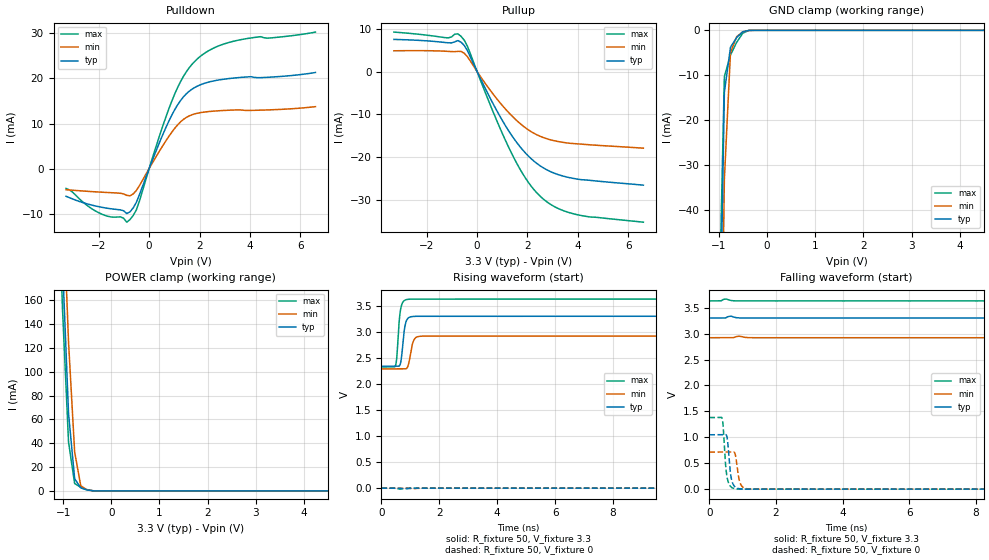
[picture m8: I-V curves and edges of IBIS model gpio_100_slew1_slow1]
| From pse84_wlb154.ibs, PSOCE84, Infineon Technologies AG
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[Model] gpio_100_slew1_slow1
Model_type I/O
Enable   Active-High
Vinl  =  0.99
Vinh  =  2.31
Vmeas =  1.65
Cref  =  15e-12
| Capacitance   typ   min   max
C_comp   1.09946e-12   1.08623e-12   1.11440e-12
| Variables   typ   min   max
[GND Clamp Reference]   0   0   0
[POWER Clamp Reference]   3.3   2.92   3.63
[Pulldown Reference]   0   0   0
[Pullup Reference]   3.3   2.92   3.63
[Temperature Range]   25   125   -40
[Voltage Range]   3.3   2.92   3.63
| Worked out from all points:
|   slope of the pulldown table from 0 to 0.495 V, typ, clamps not added: 71.6 ohm
|   slope of the pullup table from 0 to 0.495 V, typ, clamps not added: 83.3 ohm
|   GND clamp passes 1 mA (typ) near -0.57 V on its own axis
|   POWER clamp passes 1 mA (typ) near -0.52 V on its own axis
|   falling waveform, R_fixture 50, V_fixture 3.3: 20-80 % time 694ns typ, 1.01us min, 397ns max; typ from 3.3 V to 2.34 V
|   falling waveform, R_fixture 50, V_fixture 0: 20-80 % time 96.8ps typ, 105ps min, 93.7ps max; typ from 1.05 V to 0 V
|   rising waveform, R_fixture 50, V_fixture 3.3: 20-80 % time 114ps typ, 134ps min, 103ps max; typ from 2.34 V to 3.3 V
|   rising waveform, R_fixture 50, V_fixture 0: 20-80 % time 754ns typ, 1.06us min, 489ns max; typ from 0 V to 1.04 V
[GND Clamp]
| Voltage   I(typ)   I(min)   I(max)
-1.65V    -892.5mA   -911.9mA   -883.9mA
-1.015V   -92.32mA   -129.7mA   -71.28mA
-888.3mV  -13.83mA   -33.21mA   -10.31mA
-761.4mV  -3.792mA   -4.944mA   -5.509mA
-634.5mV  -1.622mA   -1.436mA   -2.707mA
-507.6mV  -326.2uA   -352.3uA   -651.6uA
-380.7mV  -13.48uA   -32.14uA   -19.55uA
-253.8mV  -189.4nA   -1.276uA   -466.7nA
6.6V      0A         0A         0A
[POWER Clamp]
| Voltage   I(typ)   I(min)   I(max)
-1.523V   838.1mA    872.9mA    823.9mA
-1.142V   346.5mA    405.1mA    310.5mA
-1.015V   193mA      257.4mA    153.9mA
-888.3mV  64.97mA    124.9mA    40.96mA
-761.4mV  10.28mA    32.7mA     6.184mA
-634.5mV  2.553mA    4.346mA    3.067mA
-507.6mV  805.9uA    960.7uA    1.159mA
-253.8mV  1.454uA    10.02uA    1.678uA
6.6V      0A         0A         0A
[Pulldown]
| Voltage   I(typ)   I(min)   I(max)
-3.3V     -6.15mA    -4.695mA   -4.423mA
-2.157V   -8.273mA   -5.161mA   -9.338mA
-1.142V   -9.173mA   -5.494mA   -10.74mA
-888.3mV  -9.988mA   -5.953mA   -11.91mA
-507.6mV  -7.509mA   -4.873mA   -9.177mA
341.4mV   4.84mA     3.249mA    6.058mA
910.3mV   11.98mA    8.158mA    15.13mA
1.366V    15.94mA    10.93mA    20.51mA
1.821V    18.03mA    12.15mA    23.86mA
2.503V    19.39mA    12.72mA    26.59mA
3.3V      20.06mA    12.98mA    28.19mA
6.6V      21.33mA    13.74mA    30.3mA
[Pullup]
| Voltage   I(typ)   I(min)   I(max)
-3.3V     7.527mA    4.862mA    9.247mA
-1.142V   6.736mA    4.723mA    7.893mA
-761.4mV  7.259mA    4.727mA    8.836mA
-634.5mV  6.867mA    4.72mA     8.248mA
-380.7mV  4.868mA    3.47mA     5.906mA
682.8mV   -8.07mA    -5.639mA   -10.11mA
1.479V    -15.86mA   -10.96mA   -20.44mA
2.048V    -19.88mA   -13.73mA   -26.08mA
2.731V    -22.92mA   -15.68mA   -30.37mA
3.3V      -24.31mA   -16.5mA    -32.32mA
4.051V    -25.28mA   -16.98mA   -33.65mA
6.6V      -26.63mA   -17.96mA   -35.32mA
[Ramp]
dV/dt_r   0.62586/0.754243u  0.420968/1.05896u  0.827993/0.488885u
dV/dt_f   0.573974/0.693875u  0.373545/1.01125u  0.781638/0.397055u
R_load = 50
[Falling Waveform]
R_fixture = 50
V_fixture = 3.3
V_fixture_min = 2.92
V_fixture_max = 3.63
| Time   V(typ)   V(min)   V(max)
0s        3.3V       2.92V      3.63V
127.1ns   3.3V       2.92V      3.598V
237.2ns   3.276V     2.92V      3.261V
319.8ns   3.185V     2.915V     3.022V
482.7ns   2.964V     2.86V      2.716V
645.6ns   2.788V     2.764V     2.553V
849.2ns   2.638V     2.653V     2.452V
1.282us   2.472V     2.492V     2.368V
1.92us    2.386V     2.378V     2.336V
4us       2.343V     2.297V     2.327V
[Falling Waveform]
R_fixture = 50
V_fixture = 0
V_fixture_min = 0
V_fixture_max = 0
| Time   V(typ)   V(min)   V(max)
0s        1.049V     715.3mV    1.381V
383.3ps   1.049V     715.1mV    1.364V
414.9ps   1.049V     715.1mV    1.21V
474.6ps   1.051V     715.2mV    568.4mV
511.4ps   1.041V     715.3mV    313.9mV
673.3ps   165mV      715.8mV    29.7mV
774.5ps   41.14mV    675mV      6.364mV
884.2ps   9.65mV     211.7mV    1.632mV
956.3ps   3.65mV     74.51mV    804.4uV
4us       19.97nV    549.4nV    10.01nV
[Rising Waveform]
R_fixture = 50
V_fixture = 3.3
V_fixture_min = 2.92
V_fixture_max = 3.63
| Time   V(typ)   V(min)   V(max)
0s        2.342V     2.29V      2.327V
480.6ps   2.341V     2.29V      2.345V
532.5ps   2.342V     2.29V      2.528V
626.9ps   2.352V     2.29V      3.285V
687ps     2.488V     2.29V      3.498V
780.9ps   3.002V     2.29V      3.598V
841.4ps   3.18V      2.291V     3.617V
931.3ps   3.268V     2.37V      3.626V
1.119ns   3.297V     2.841V     3.629V
4us       3.3V       2.92V      3.63V
[Rising Waveform]
R_fixture = 50
V_fixture = 0
V_fixture_min = 0
V_fixture_max = 0
| Time   V(typ)   V(min)   V(max)
0s        17.41nV    537.5nV    10.27nV
146.4ns   1.058mV    143.2uV    59.16mV
253.4ns   43.81mV    2.628mV    320.9mV
375.7ns   175.3mV    25.9mV     624mV
579.3ns   422.5mV    121mV      966.7mV
742.2ns   585.6mV    213.1mV    1.116V
945.9ns   734.1mV    320.8mV    1.215V
1.357us   895mV      483.4mV    1.308V
1.988us   985.6mV    611mV      1.358V
4us       1.043V     701.6mV    1.38V
